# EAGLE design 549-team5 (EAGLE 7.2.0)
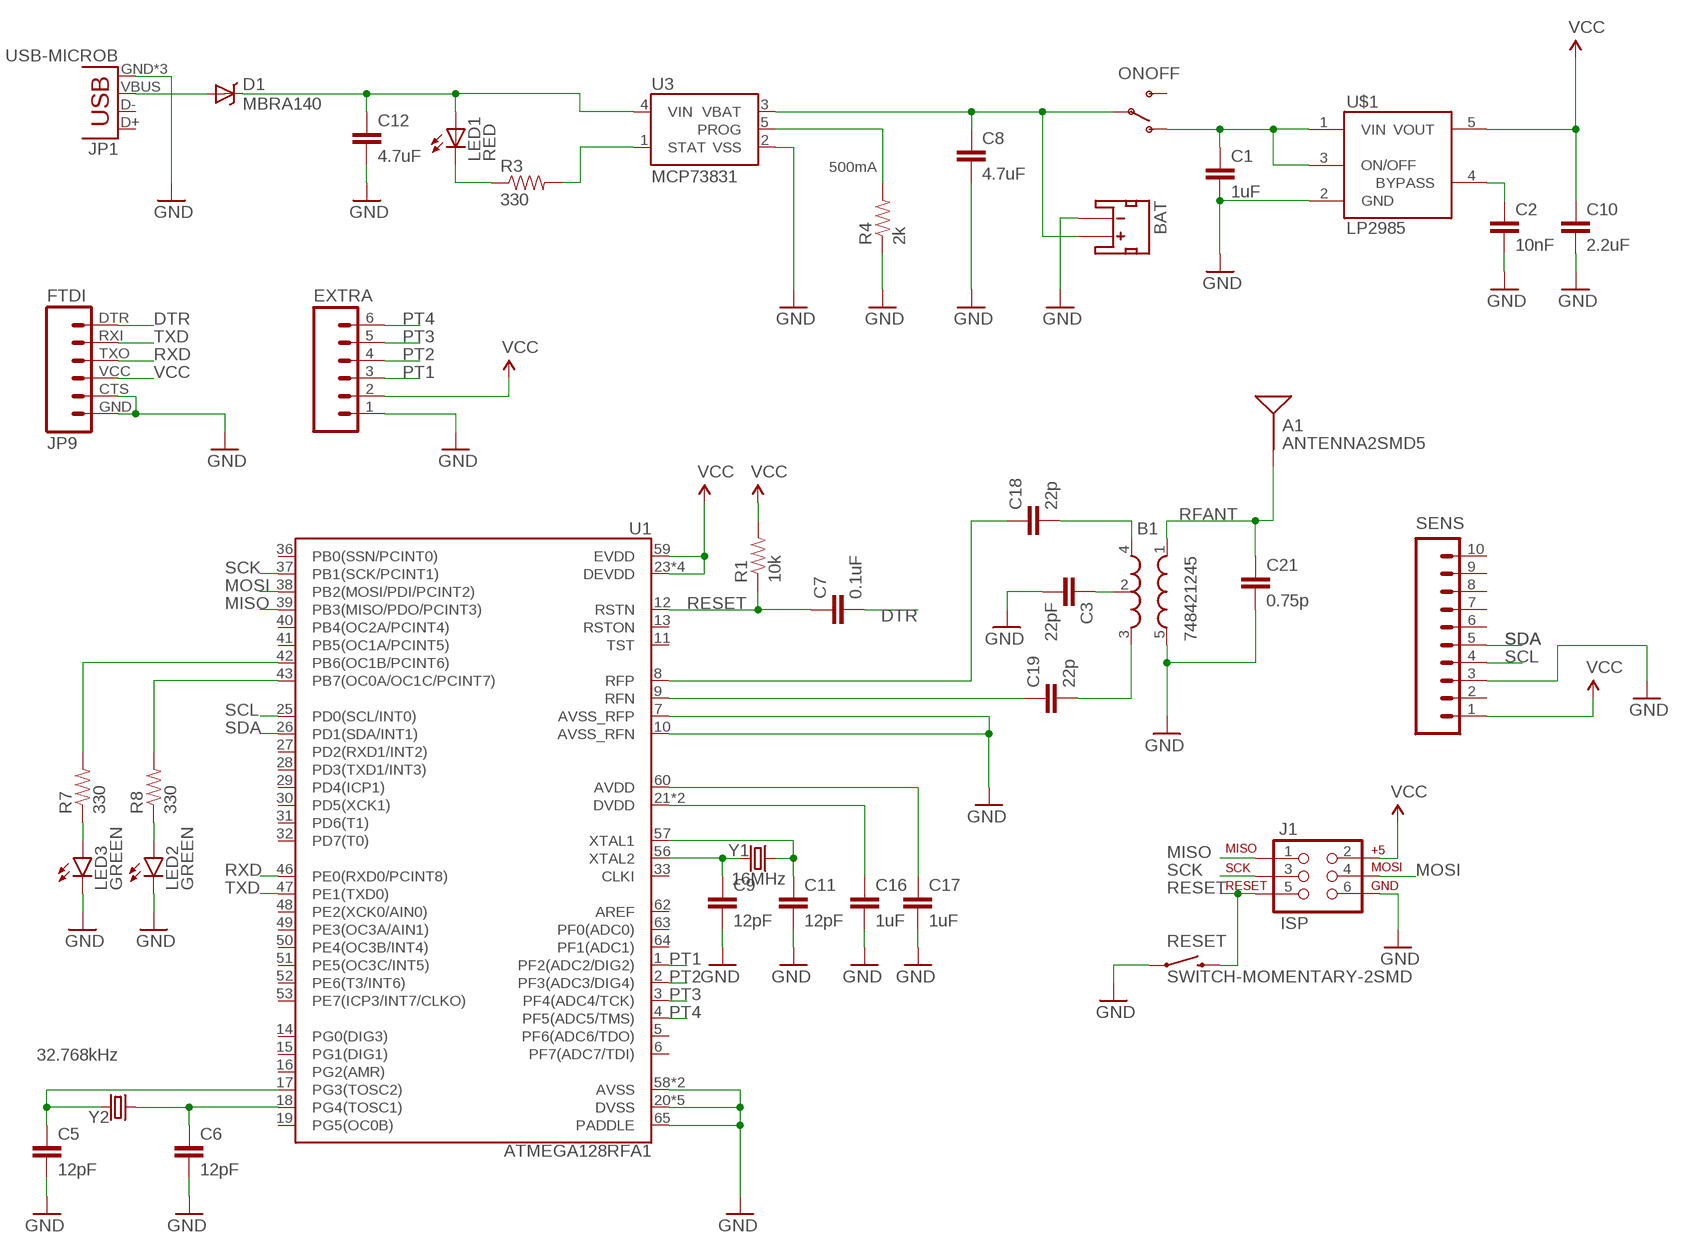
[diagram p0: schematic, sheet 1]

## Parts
A1  ANTENNA2SMD5  [ANTENNA-CHIP5]
B1  748421245  BALUN0805  [BALUN]
BAT  JST_2MM_MALE  [JST-2-SMD]
C1  1uF  CAP1206  [1206]
C2  10nF  CAP1206  [1206]
C3  22pF  CAP1206  [1206]
C5  12pF  CAP1206  [1206]
C6  12pF  CAP1206  [1206]
C7  0.1uF  CAP1206  [1206]
C8  4.7uF  CAP1206  [1206]
C9  12pF  CAP1206  [1206]
C10  2.2uF  CAP1206  [1206]
C11  12pF  CAP1206  [1206]
C12  4.7uF  CAP1206  [1206]
C16  1uF  CAP1206  [1206]
C17  1uF  CAP1206  [1206]
C18  22p  CAP1206  [1206]
C19  22p  CAP1206  [1206]
C21  0.75p  CAP1206  [1206]
D1  MBRA140  [SMA-DIODE]
EXTRA  M06SILK_FEMALE_PTH  [1X06]
J1  ISP  AVR_SPI_PRG_6NS  [2X3-NS]
JP1  USB-MICROB  [USB-MICROB]
JP9  FTDI  FTDI_BASICPTH  [FTDI_BASIC]
LED1  RED  LED1206  [LED-1206]
LED2  GREEN  LED1206  [LED-1206]
LED3  GREEN  LED1206  [LED-1206]
ONOFF  SWITCH-SPST-SMD-A  [SWITCH-SPST-SMD-A]
R1  10k  RESISTOR1206  [1206]
R3  330  RESISTOR1206  [1206]
R4  2k  RESISTOR1206  [1206]
R7  330  RESISTOR1206  [1206]
R8  330  RESISTOR1206  [1206]
RESET  SWITCH-MOMENTARY-2SMD  [TACTILE-SWITCH-SMD]
SENS  M10SILK_FEMALE_PTH  [1X10]
U1  ATMEGA128RFA1  [QFN-64]
U3  MCP73831  [SOT23-5]
U$1  LP2985AIM5-3.3  [SOT25]
Y1  16MHz  CRYSTAL5X3  [CRYSTAL-SMD-5X3]
Y2  32.768kHz  CRYSTAL32-SMD  [CRYSTAL-32KHZ-SMD]

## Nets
AVDD: C17.1 U1.60(AVDD)
BYPASS: C2.1 U$1.4(BYPASS)
DTR: C7.2 JP9.DTR
DVDD: C16.1 U1.21(DVDD) U1.22(DVDD)
GND: B1.5(GND) BAT.1(-) C1.2 C2.2 C3.2 C5.2 C6.2 C8.2 C9.2 C10.2 C11.2 C12.2 C16.2 C17.2 C21.2 EXTRA.1 J1.6 JP1.GND JP1.MT1(GND) JP1.MT2(GND) JP9.CTS JP9.GND LED2.C LED3.C R4.1 RESET.1 SENS.3 U1.7(AVSS_RFP) U1.10(AVSS_RFN) U1.20(DVSS) U1.24(DVSS) U1.35(DVSS) U1.45(DVSS) U1.55(DVSS) U1.58(AVSS) U1.61(AVSS) U1.65(PADDLE) U3.2(VSS) U$1.2(GND)
MISO: J1.1 U1.39(PB3(MISO/PDO/PCINT3))
MOSI: J1.4 U1.38(PB2(MOSI/PDI/PCINT2))
N$1: R8.2 U1.43(PB7(OC0A/OC1C/PCINT7))
N$3: C11.1 U1.57(XTAL1) Y1.3
N$4: C9.1 U1.56(XTAL2) Y1.1
N$5: C6.1 U1.18(PG4(TOSC1)) Y2.X1
N$6: C5.1 U1.17(PG3(TOSC2)) Y2.X2
N$7: C1.1 ONOFF.1(O) U$1.1(VIN) U$1.3(ON/OFF)
N$8: LED3.A R7.1
N$9: BAT.2(+) C8.1 ONOFF.2(P) U3.3(VBAT)
N$10: B1.4(OUT1) C18.2
N$11: B1.3(OUT2) C19.2
N$12: R7.2 U1.42(PB6(OC1B/PCINT6))
N$13: LED2.A R8.1
N$14: B1.2(GND) C3.1
N$15: C12.1 D1.C LED1.A U3.4(VIN)
N$18: R3.2 U3.1(STAT)
N$19: LED1.C R3.1
N$20: D1.A JP1.VBUS
PROG: R4.2 U3.5(PROG)
PT1: EXTRA.3 U1.1(PF2(ADC2/DIG2))
PT2: EXTRA.4 U1.2(PF3(ADC3/DIG4))
PT3: EXTRA.5 U1.3(PF4(ADC4/TCK))
PT4: EXTRA.6 U1.4(PF5(ADC5/TMS))
RESET: C7.1 J1.5 R1.1 RESET.3 U1.12(RSTN)
RFANT: A1.FEED(SIGNAL) B1.1(IN) C21.1
RFN: C19.1 U1.9(RFN)
RFP: C18.1 U1.8(RFP)
RXD: JP9.TXO U1.46(PE0(RXD0/PCINT8))
SCK: J1.3 U1.37(PB1(SCK/PCINT1))
SCL: SENS.4 U1.25(PD0(SCL/INT0))
SDA: SENS.5 U1.26(PD1(SDA/INT1))
TXD: JP9.RXI U1.47(PE1(TXD0))
VCC: C10.1 EXTRA.2 J1.2 JP9.VCC R1.2 SENS.1 U1.23(DEVDD) U1.34(DEVDD) U1.44(DEVDD) U1.54(DEVDD) U1.59(EVDD) U$1.5(VOUT)
Unconnected: BAT.NC1(PAD1) BAT.NC2(PAD2) JP1.D+ JP1.D- ONOFF.3(S) SENS.2 SENS.6 SENS.7 SENS.8 SENS.9 SENS.10 U1.5(PF6(ADC6/TDO)) U1.6(PF7(ADC7/TDI)) U1.11(TST) U1.13(RSTON) U1.14(PG0(DIG3)) U1.15(PG1(DIG1)) U1.16(PG2(AMR)) U1.19(PG5(OC0B)) U1.27(PD2(RXD1/INT2)) U1.28(PD3(TXD1/INT3)) U1.29(PD4(ICP1)) U1.30(PD5(XCK1)) U1.31(PD6(T1)) U1.32(PD7(T0)) U1.33(CLKI) U1.36(PB0(SSN/PCINT0)) U1.40(PB4(OC2A/PCINT4)) U1.41(PB5(OC1A/PCINT5)) U1.48(PE2(XCK0/AIN0)) U1.49(PE3(OC3A/AIN1)) U1.50(PE4(OC3B/INT4)) U1.51(PE5(OC3C/INT5)) U1.52(PE6(T3/INT6)) U1.53(PE7(ICP3/INT7/CLKO)) U1.62(AREF) U1.63(PF0(ADC0)) U1.64(PF1(ADC1))

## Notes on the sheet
- 500mA

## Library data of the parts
A1 = SparkFun-RF:ANTENNA2: Chip antenna
B1 = SparkFun-RF:BALUN: 0805 footprint balun- Ember 351/357
BAT = SparkFun-Connectors:JST_2MM_MALE: Mates to single-cell LiPo batteries. CONN-08352; PROD_ID: CONN-08352
C1-C3 C5-C12 C16-C19 C21 = SparkFun-Capacitors:CAP: Capacitor
D1 = SparkFun-DiscreteSemi:MBRA140: 40V, 1A Schottky rectifier; PROD_ID: DIO-08053
EXTRA = SparkFun-Connectors:M06: Header 6 Standard 6-pin 0.1" header. Use with straight break away headers (SKU : PRT-00116), right angle break away headers (PRT-00553), swiss pins (PRT-00743), machine pins (PRT-00117), and female headers (PRT-00115). Molex polarized connector foot print use with SKU : PRT-08094 with associated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; PROD_ID: CONN-08437
J1 = SparkFun-Connectors:AVR_SPI_PRG_6: AVR ISP 6 Pin This is the reduced ISP connector for AVR programming. Common on Arduino. This footprint will take up less PCB space and can be used with a 10-pin to 6-pin adapter such as SKU: BOB-08508
JP1 = SparkFun-Connectors:USB: USB Connectors USB-B-PTH is fully proven SKU : PRT-00139/CONN-08278 USB-miniB is fully proven SKU : PRT-00587 USB-A-PCB is untested. USB-A-H is throughly reviewed, but untested. Spark Fun Electronics SKU : PRT-00437 USB-B-SMT is throughly reviewed, but untested. Needs silkscreen touching up.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; PROD_ID: CONN-09505
JP9 = SparkFun-Connectors:FTDI_BASIC: FTDI Basic header with labels
LED1 = LilyPad-Wearables:LED: LEDs
LED2 LED3 = SparkFun-LED:LED: LEDs
ONOFF = SparkFun:SWITCH-SPST: SPST Switch Simple slide switch. Spark Fun Electronics SKU : COM-00102
R1 R3 R4 R7 R8 = SparkFun-Passives:RESISTOR: Resistor
RESET = SparkFun-Electromechanical:SWITCH-MOMENTARY-2: Various NO switches- pushbuttons, reed, etc; PROD_ID: SWCH-08247
SENS = SparkFun-Connectors:M10: Header 10 Standard 10-pin 0.1" header. Use with straight break away headers (SKU : PRT-00116), right angle break away headers (PRT-00553), swiss pins (PRT-00743), machine pins (PRT-00117), and female headers (PRT-00115).; PROD_ID: CONN-11563
U1 = SparkFun-DigitalIC:ATMEGA128RFA1: ATmega128RFA1 8-bit AVR Microcontroller with Low Power 2.4GHz Transceiver for ZigBee and IEEE 802.15.4
U3 = SparkFun-PowerIC:MCP73831: Miniature single cell, fully integrated Li-Ion, Li-polymer charge management controller http://ww1.microchip.com/downloads/en/DeviceDoc/21984a.pdf IC-09995; PROD_ID: IC-09995
U$1 = LP2985:LP2985: LP2985-N Micropower 150 mA Low-Noise Ultra Low-Dropout Regulator
Y1 Y2 = SparkFun-FreqCtrl:CRYSTAL: Various standard crystals. Proven footprints. Spark Fun Electronics SKU : COM-00534

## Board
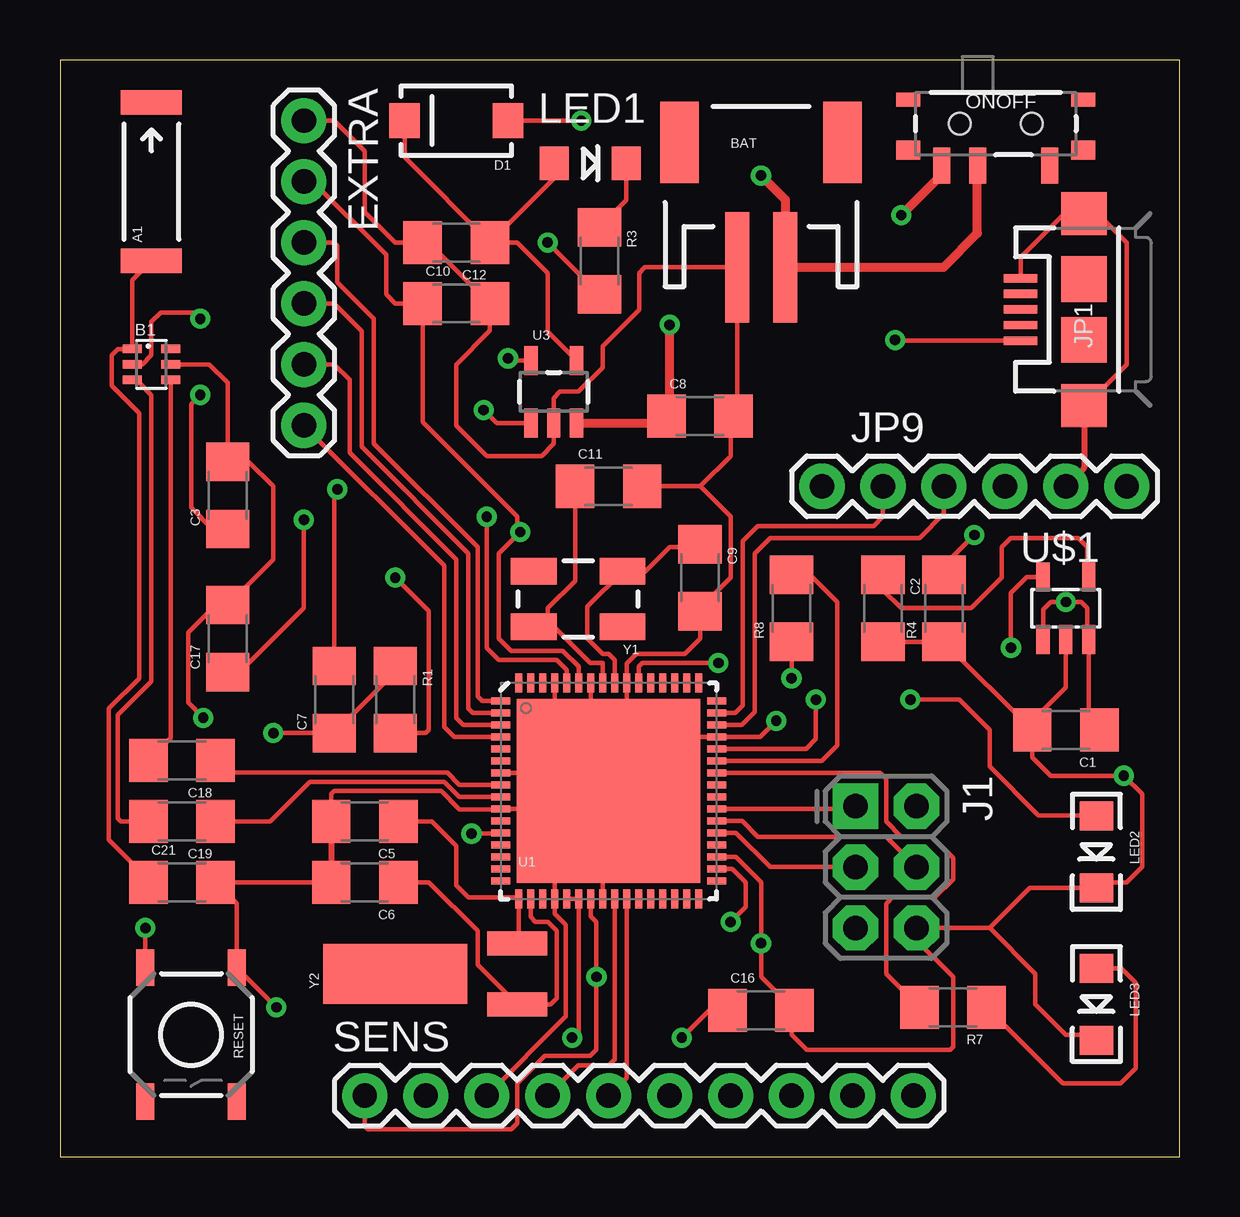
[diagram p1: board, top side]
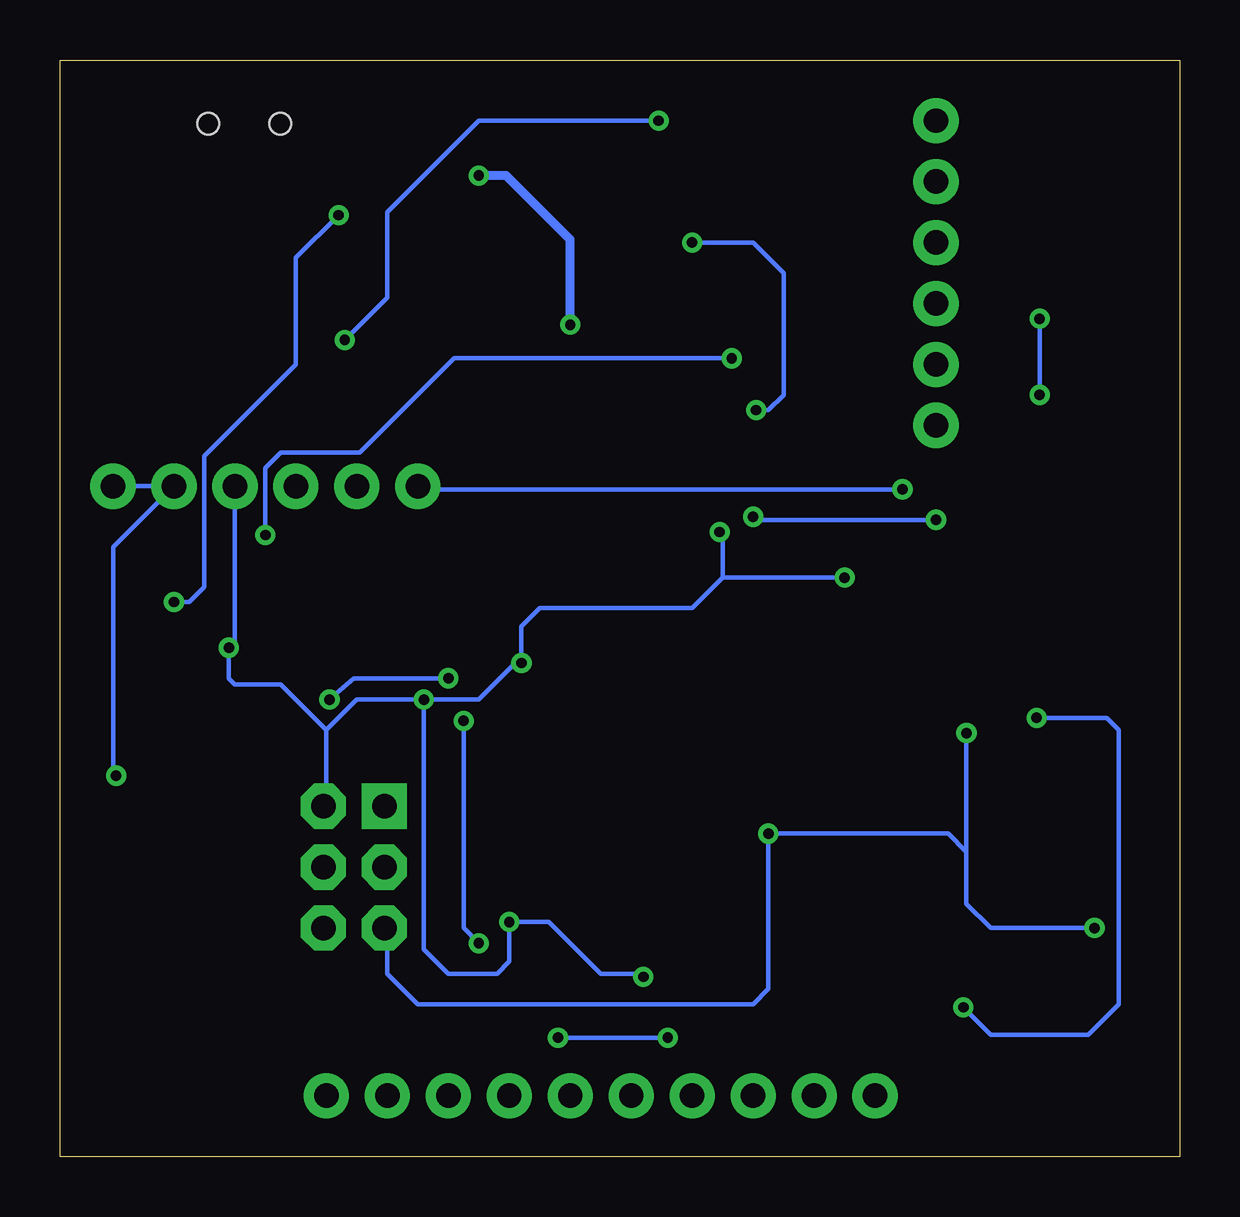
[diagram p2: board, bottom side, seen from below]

Size 46.66 x 45.71 mm. Coordinates in mm from the lower left corner, seen from the top.
Outline: 0,0 46.66,0 46.66,45.71 0,45.71 0,0
Copper layers (1*16): Top 0.035mm / dielectric 1.5mm / Bottom 0.035mm
Design rules "default *": minimum track width 7mil, minimum drill 16mil, track to track 7mil, track to pad 7mil, pad to pad 7mil, via to via 7mil, smd to smd 7mil, copper to edge 40mil, drill to drill 7mil, minimum pad ring 10mil, minimum via ring 8mil, stop-mask expansion 4mil, vias tented up to drill 0mil, thermal gap 10mil

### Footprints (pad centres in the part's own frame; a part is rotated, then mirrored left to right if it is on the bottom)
ANTENNA-CHIP5 = smd 1.016 x 2.54: FEED -3.302,0; NC 3.302,0
BALUN = smd 0.35 x 0.8: 1 -0.65,-0.8; 2 0,-0.8; 3 0.65,-0.8; 4 0.65,0.8; 5 0,0.8; 6 -0.65,0.8
JST-2-SMD = smd 1 x 4.6: 1 -1,-3.7; 2 1,-3.7 | smd 1.6 x 3.4: NC1 -3.4,1.5; NC2 3.4,1.5
1206 = smd 1.6 x 1.8: 1 -1.4,0; 2 1.4,0
SMA-DIODE = smd 1.27 x 1.47: A -2.15,0; C 2.15,0
1X06 = drill 1.016 pad 1.88: 1 0,0; 2 2.54,0; 3 5.08,0; 4 7.62,0; 5 10.16,0; 6 12.7,0
2X3-NS = drill 1.016 pad 1.88 square: 1 -2.54,-1.27 | drill 1.016 pad 1.88 octagon: 2 -2.54,1.27; 3 0,-1.27; 4 0,1.27; 5 2.54,-1.27; 6 2.54,1.27
USB-MICROB = smd 0.35 x 1.4: D+ 0,2.65; D- -0.65,2.65; GND 1.3,2.65; ID 0.65,2.65; VBUS -1.3,2.65 | smd 1.8 x 1.9: MT1 -4,0; MT2 4,0 | smd 1.9 x 1.9: P$1 -1.27,0; P$2 1.27,0
FTDI_BASIC = drill 1.016 pad 1.88: CTS 10.16,0; DTR 0,0; GND 12.7,0; RXI 2.54,0; TXO 5.08,0; VCC 7.62,0
LED-1206 = smd 1.2 x 1.4: A -1.5,0; C 1.5,0
SWITCH-SPST-SMD-A = smd 0.7 x 1.5: 1 -2.25,-1.75; 2 -0.75,-1.75; 3 2.25,-1.75 | smd 1 x 0.6: GND1 -3.65,1; GND3 3.65,1 | smd 1 x 0.8: GND2 -3.65,-1.1; GND4 3.65,-1.1 | hole 0.9: -1.5,0; 1.5,0
TACTILE-SWITCH-SMD = smd 1.524 x 0.762: 1 -2.794,1.905; 2 2.794,1.905; 3 -2.794,-1.905; 4 2.794,-1.905
1X10 = drill 1.016 pad 1.88: 1 0,0; 2 2.54,0; 3 5.08,0; 4 7.62,0; 5 10.16,0; 6 12.7,0; 7 15.24,0; 8 17.78,0; 9 20.32,0; 10 22.86,0
QFN-64 = smd 0.8 x 0.28: 1 -4.5,3.75; 2 -4.5,3.25; 3 -4.5,2.75; 4 -4.5,2.25; 5 -4.5,1.75; 6 -4.5,1.25; 7 -4.5,0.75; 8 -4.5,0.25; 9 -4.5,-0.25; 10 -4.5,-0.75; 11 -4.5,-1.25; 12 -4.5,-1.75; 13 -4.5,-2.25; 14 -4.5,-2.75; 15 -4.5,-3.25; 16 -4.5,-3.75; 33 4.5,-3.75; 34 4.5,-3.25; 35 4.5,-2.75; 36 4.5,-2.25; 37 4.5,-1.75; 38 4.5,-1.25; 39 4.5,-0.75; 40 4.5,-0.25; 41 4.5,0.25; 42 4.5,0.75; 43 4.5,1.25; 44 4.5,1.75; 45 4.5,2.25; 46 4.5,2.75; 47 4.5,3.25; 48 4.5,3.75 | smd 0.28 x 0.8: 17 -3.75,-4.5; 18 -3.25,-4.5; 19 -2.75,-4.5; 20 -2.25,-4.5; 21 -1.75,-4.5; 22 -1.25,-4.5; 23 -0.75,-4.5; 24 -0.25,-4.5; 25 0.25,-4.5; 26 0.75,-4.5; 27 1.25,-4.5; 28 1.75,-4.5; 29 2.25,-4.5; 30 2.75,-4.5; 31 3.25,-4.5; 32 3.75,-4.5; 49 3.75,4.5; 50 3.25,4.5; 51 2.75,4.5; 52 2.25,4.5; 53 1.75,4.5; 54 1.25,4.5; 55 0.75,4.5; 56 0.25,4.5; 57 -0.25,4.5; 58 -0.75,4.5; 59 -1.25,4.5; 60 -1.75,4.5; 61 -2.25,4.5; 62 -2.75,4.5; 63 -3.25,4.5; 64 -3.75,4.5 | smd 7.65 x 7.65: 65 0,0
SOT23-5 = smd 0.55 x 1.2: 1 -0.95,-1.3; 2 0,-1.3; 3 0.95,-1.3; 4 0.95,1.3; 5 -0.95,1.3
SOT25 = smd 0.55 x 1.2: 1 -0.95,-1.3; 2 0,-1.3; 3 0.95,-1.3; 4 0.95,1.3; 5 -0.95,1.3
CRYSTAL-SMD-5X3 = smd 1.9 x 1.1: 1 -1.85,-1.15; 2 1.85,-1.15; 3 1.85,1.15; 4 -1.85,1.15
CRYSTAL-32KHZ-SMD = smd 2.5 x 6: SHEILD 0,5.08 | smd 1 x 2.5: X1 -1.27,0; X2 1.27,0

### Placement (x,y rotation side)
A1  3.81,40.64 90 top
B1  3.81,33.02 270 top
BAT  29.21,40.77 0 top
C1  41.91,17.78 180 top
C2  34.29,22.86 270 top
C3  6.99,27.56 90 top
C5  12.7,13.97 180 top
C6  12.7,11.43 180 top
C7  11.43,19.05 90 top
C8  26.67,30.86 0 top
C9  26.67,24.13 270 top
C10  16.51,35.56 0 top
C11  22.86,27.94 0 top
C12  16.51,38.1 180 top
C16  29.21,6.1 0 top
C17  6.99,21.59 90 top
C18  5.08,16.51 180 top
C19  5.08,13.97 180 top
C21  5.08,11.43 0 top
D1  16.51,43.18 180 top
EXTRA  10.16,43.18 270 top
J1  34.42,12.06 270 top
JP1  42.67,35.31 90 top
JP9  31.75,27.94 0 top
LED1  22.1,41.4 0 top
LED2  43.18,12.7 270 top
LED3  43.18,6.35 270 top
ONOFF  38.99,43.05 0 top
R1  13.97,19.05 270 top
R3  22.48,37.34 270 top
R4  36.83,22.86 90 top
R7  37.21,6.22 180 top
R8  30.48,22.86 90 top
RESET  5.46,5.08 270 top
SENS  12.7,2.54 0 top
U1  22.86,15.24 0 top
U3  20.57,31.88 0 top
U$1  41.91,22.86 0 top
Y1  21.59,23.24 180 top
Y2  19.05,7.62 90 top

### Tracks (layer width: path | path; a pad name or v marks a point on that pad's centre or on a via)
AVDD  (via drill 0.43)
  Top 0.178: U1.60 21.11,20.29 20.7,20.7 18.29,20.7 17.78,21.21 v17.78,26.67 | C17.1 7.49,20.19 10.16,22.86 v10.16,26.54
  Bottom 0.178: v10.16,26.54 17.65,26.54 v17.78,26.67
BYPASS
  Top 0.178: C2.1 34.29,23.62 35.05,22.86 37.97,22.86 39.24,24.13 39.24,25.4 39.62,25.78 42.42,25.78 42.8,25.4 42.8,24.22 U$1.4
DTR  (via drill 0.43)
  Top 0.178: C7.2 11.43,27.69 v11.56,27.81
  Bottom 0.178: v11.56,27.81 31.62,27.81 JP9.DTR
DVDD  (via drill 0.43)
  Top 0.178: U1.21 U1.22 21.61,5.23 v21.34,4.95 | C16.1 27.05,6.1 v25.91,4.95
  Bottom 0.178: v21.34,4.95 v25.91,4.95
GND  (via drill 0.43)
  Top 0.178: SENS.3 21.08,5.84 21.08,9.65 20.61,10.12 U1.20 20.61,15.24 | U1.35 28.15,12.49 29.21,11.43 v29.21,8.89 29.21,7.5 C16.2 30.48,5.97 30.48,5.08 31.11,4.45 37.08,4.45 37.21,4.57 37.21,7.49 35.69,9.02 J1.6 38.73,9.53 | 38.73,9.53 40.64,7.62 40.64,6.35 41.91,5.08 42.95,5.08 LED3.C | U1.7 20.32,15.99 | 20.32,15.99 21.59,15.99 | 21.59,15.99 22.11,15.99 U1.65 22.61,14.99 U1.24 | U1.58 22.11,17.78 | 22.11,17.78 22.11,16.51 21.59,15.99 | U1.61 20.61,16.28 20.32,15.99 | 23.61,18.53 U1.55 23.61,20.56 24,20.95 26.04,20.95 26.67,21.59 C9.2 26.67,22.86 27.94,24.13 27.94,26.67 26.67,27.94 | 23.61,18.53 22.86,17.78 22.11,17.78 | 23.61,18.53 24.65,17.49 U1.45 29.17,17.49 v29.84,18.16 | 20.61,15.24 20.61,15.7 20.32,15.99 | 20.61,15.24 19.86,14.49 U1.10 18.35,14.48 16.64,14.48 15.88,15.24 11.43,15.24 11.3,15.11 C5.2 | C6.2 C21.2 7.37,10.54 RESET.1 v9.02,6.22 | B1.5 6.22,33.02 6.99,32.26 C3.2 7.87,28.96 8.89,27.94 8.89,24.89 C17.2 6.48,22.99 5.33,21.84 5.33,18.92 v5.97,18.29 | 38.73,9.53 40.41,11.2 LED2.C 43.41,11.43 44.45,11.43 45.09,12.06 45.09,15.11 v44.32,15.88 41.27,15.88 40.51,16.64 C1.2 | U$1.2 41.91,19.56 40.64,18.29 40.64,17.91 C1.2 | EXTRA.1 11.43,43.18 12.7,41.91 12.7,39.37 13.97,38.1 C12.2 15.37,38.1 C10.2 17.91,34.42 16.51,33.02 16.51,30.48 17.78,29.21 20.07,29.21 20.57,29.72 U3.2 20.57,31.62 20.83,31.88 21.59,31.88 22.61,32.89 22.61,33.78 24.13,35.31 24.13,36.83 24.37,37.07 BAT.1 28.21,31 C8.2 27.94,30.73 27.94,29.21 26.67,27.94 | C2.2 R4.1 C1.2 | C11.2 26.67,27.94 | JP1.GND 40.02,37.48 41.91,39.37 42.61,39.37 JP1.MT2 42.74,39.37 43.18,39.37 44.45,38.1 44.45,33.02 42.74,31.31 JP1.MT1
  Top 0.254: C5.2 C6.2 | JP1.MT1 42.67,28.7 JP9.CTS | JP1.MT2 42.67,39.26
  Bottom 0.178: v5.97,18.29 3.05,18.29 2.54,17.78 2.54,6.35 3.81,5.08 7.87,5.08 v9.02,6.22 | JP9.GND JP9.CTS 44.45,25.4 44.45,16 v44.32,15.88 | v29.84,18.16 29.84,9.53 v29.21,8.89
MISO
  Top 0.178: U1.39 33.03,14.49 J1.1
MOSI
  Top 0.178: U1.38 28.43,13.99 29.08,13.34 34.42,13.34 J1.4
N$1
  Top 0.178: U1.43 31.73,16.49 32.38,17.14 32.38,23.11 31.37,24.13 30.61,24.13 R8.2
N$3
  Top 0.178: 20.32,22.1 20.57,22.1 22.1,20.57 22.61,20.57 U1.57 | 20.32,22.1 Y1.3 | C11.1 21.46,24 20.32,22.86 20.32,22.1
N$4
  Top 0.178: C9.1 26.54,25.4 25.4,25.4 24.39,24.39 Y1.1 21.97,22.92 21.97,21.59 22.61,20.95 22.86,20.95 23.11,20.7 U1.56
N$5
  Top 0.178: U1.18 19.61,9.98 19.81,9.78 20.32,9.78 20.7,9.4 20.7,6.6 20.45,6.35 Y2.X1 17.4,8 17.4,9.4 15.37,11.43 C6.1
N$6
  Top 0.178: Y2.X2 19.11,8.95 U1.17 19.05,10.79 17.02,10.79 16.51,11.3 16.51,12.95 15.49,13.97 C5.1 13.97,13.97
N$7  (via drill 0.43)
  Top 0.178: C1.1 42.86,18.23 U$1.3 42.8,21.62 42.8,22.86 42.55,23.11 v41.91,23.11 41.27,23.11 40.96,22.8 U$1.1 | ONOFF.1 36.74,40.93
  Top 0.381: 36.74,40.93 v35.05,39.24
  Bottom 0.178: v41.91,23.11 41.27,23.11 40.64,23.75 40.64,29.21 36.83,33.02 36.83,37.47 v35.05,39.24
N$8
  Top 0.178: LED3.A 44.22,7.85 44.83,7.24 44.83,3.68 44.2,3.05 41.79,3.05 R7.1
N$9  (via drill 0.43)
  Top 0.178: 25.4,30.99 C8.1 | 38.1,41.16 ONOFF.2
  Top 0.381: U3.3 24.99,30.58 C8.1 | 25.4,30.99 v25.4,34.67 | v29.21,40.89 30.23,39.88 30.23,37.08 BAT.2 36.81,37.07 38.23,38.48 38.23,41.29 ONOFF.2
  Top 0.508: 25.27,30.58 C8.1 | v25.4,34.67 25.27,34.67
  Bottom 0.381: v25.4,34.67 25.4,38.23 28.07,40.89 v29.21,40.89
N$10
  Top 0.178: B1.4 4.61,17.44 C18.2
N$11
  Top 0.178: B1.3 3.19,32.37 3.81,31.75 3.81,19.81 2.41,18.41 2.41,14.1 2.54,13.97 C19.2
N$12
  Top 0.178: U1.42 34.17,15.99 34.42,15.75 34.42,13.97 35.05,13.34 36.32,13.34 37.21,12.45 37.21,11.56 36.45,10.79 34.67,10.79 34.42,10.54 34.42,7.62 R7.2
N$13  (via drill 0.43)
  Top 0.178: R8.1 v30.48,19.94 | v35.43,19.05 37.47,19.05 38.73,17.78 38.73,16.26 40.77,14.22 43.16,14.22 LED2.A
  Bottom 0.178: v30.48,19.94 34.42,19.94 v35.43,19.05
N$14  (via drill 0.43)
  Top 0.178: C3.1 6.35,26.16 5.46,27.05 5.46,31.37 v5.84,31.75 | B1.2 3.43,33.02 3.81,33.4 3.81,34.8 4.19,35.18 5.59,35.18 v5.84,34.92
  Bottom 0.178: v5.84,34.92 v5.84,31.75
N$15
  Top 0.178: D1.C 14.36,41.65 C12.1 | LED1.A 20.6,40.79 C12.1 | C12.1 19.05,38.1 20.32,36.83 20.32,34.38 U3.4
N$18  (via drill 0.43)
  Top 0.178: R3.2 v20.32,38.1 | U3.1 18.19,30.58 v17.65,31.11
  Bottom 0.178: v17.65,31.11 17.14,31.11 16.51,31.75 16.51,36.83 17.78,38.1 v20.32,38.1
N$19
  Top 0.178: LED1.C 23.6,39.86 R3.1
N$20  (via drill 0.43)
  Top 0.178: D1.A v21.72,43.18 | JP1.VBUS 34.83,34.01 v34.8,34.04
  Bottom 0.178: v21.72,43.18 29.21,43.18 33.02,39.37 33.02,35.81 v34.8,34.04
PROG  (via drill 0.43)
  Top 0.178: R4.2 36.83,24.64 v38.1,25.91 | U3.5 18.77,33.18 v18.67,33.27
  Bottom 0.178: v38.1,25.91 38.1,28.7 37.47,29.34 34.16,29.34 30.23,33.27 v18.67,33.27
PT1
  Top 0.178: U1.1 17.59,18.99 17.4,19.18 17.4,25.4 13.08,29.72 13.08,34.92 11.56,36.45 11.56,37.97 11.43,38.1 EXTRA.3
PT2
  Top 0.178: U1.2 17.2,18.49 17.02,18.67 17.02,25.15 12.57,29.59 12.57,34.42 11.43,35.56 EXTRA.4
PT3
  Top 0.178: U1.3 16.81,17.99 16.51,18.29 16.51,24.89 12.06,29.34 12.06,32.38 11.43,33.02 EXTRA.5
PT4
  Top 0.178: U1.4 16.42,17.49 16,17.91 16,24.64 EXTRA.6
RESET  (via drill 0.43)
  Top 0.178: v17.14,13.46 18.33,13.46 U1.12 | RESET.3 v3.56,9.53 | R1.1 13.97,20.19 C7.1 v8.89,17.65
  Bottom 0.178: v8.89,17.65 8.89,12.7 | 8.89,12.7 8.89,10.54 7.87,9.53 v3.56,9.53 | 8.89,12.7 9.65,13.46 v17.14,13.46 17.14,6.99 17.78,6.35 31.75,6.35 33.02,7.62 33.02,9.4 J1.5
RFANT
  Top 0.178: 3.81,11.43 C21.1 3.68,11.56 2.03,13.21 2.03,18.67 3.3,19.94 3.3,30.99 2.16,32.13 2.16,33.4 2.41,33.66 3,33.66 B1.1 3.01,36.54 A1.FEED
RFN
  Top 0.178: U1.9 16.63,14.99 16,15.62 10.41,15.62 8.76,13.97 C19.1
RFP
  Top 0.178: U1.8 16.64,15.49 16.13,16 6.99,16 C18.1
RXD
  Top 0.178: U1.46 28.4,17.99 28.96,18.54 28.96,25.15 29.59,25.78 35.81,25.78 36.83,26.8 JP9.TXO
SCK
  Top 0.178: U1.37 28.17,13.49 29.59,12.06 J1.3
SCL
  Top 0.178: U1.25 23.11,4.06 22.86,3.81 21.59,3.81 SENS.4
SDA
  Top 0.178: U1.26 23.61,3.29 SENS.5
TXD
  Top 0.178: U1.47 28.14,18.49 28.45,18.8 28.45,25.65 29.08,26.29 33.91,26.29 34.29,26.67 JP9.RXI
VCC  (via drill 0.43)
  Top 0.178: SENS.1 12.7,1.27 12.83,1.14 18.8,1.14 19.05,1.4 19.05,3.05 20.19,4.19 22.1,4.19 22.35,4.45 v22.35,7.49 22.35,9.78 22.11,10.02 U1.23 | EXTRA.2 10.54,40.64 13.59,37.59 13.59,35.94 13.97,35.56 C10.1 15.11,30.61 19.05,26.67 19.05,26.16 v19.18,26.04 18.29,25.15 18.29,21.59 18.8,21.08 20.95,21.08 21.61,20.43 U1.59 | U1.54 24.11,20.43 24.26,20.57 v27.43,20.57 | U1.34 28.02,11.99 28.57,11.43 28.57,10.41 v27.94,9.78 | U1.44 31.09,16.99 31.5,17.4 v31.5,19.05 | U$1.5 40.29,24.16 39.62,23.5 v39.62,21.21 | R1.2 15.24,17.65 15.37,17.78 15.37,22.73 v13.97,24.13
  Bottom 0.178: 19.05,24.13 20.32,22.86 26.67,22.86 27.43,22.1 v27.43,20.57 27.69,20.57 29.21,19.05 v31.5,19.05 | 19.05,24.13 19.05,25.91 v19.18,26.04 | v31.5,19.05 34.29,19.05 35.56,17.78 | 35.56,17.78 35.56,14.73 J1.2 | v22.35,7.49 22.48,7.62 24.13,7.62 26.29,9.78 v27.94,9.78 27.94,8.13 28.45,7.62 30.48,7.62 31.5,8.64 v31.5,19.05 | 35.56,17.78 37.47,19.68 39.37,19.68 39.62,19.94 v39.62,21.21 39.37,21.46 JP9.VCC | v13.97,24.13 19.05,24.13

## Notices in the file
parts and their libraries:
SparkFun-Aesthetics: Licensing: CC v3.0 Share-Alike You are welcome to use this library for commercial purposes.
SparkFun-Capacitors: Licensing: Creative Commons ShareAlike 4.0 International - https://creativecommons.org/licenses/by-sa/4.0
